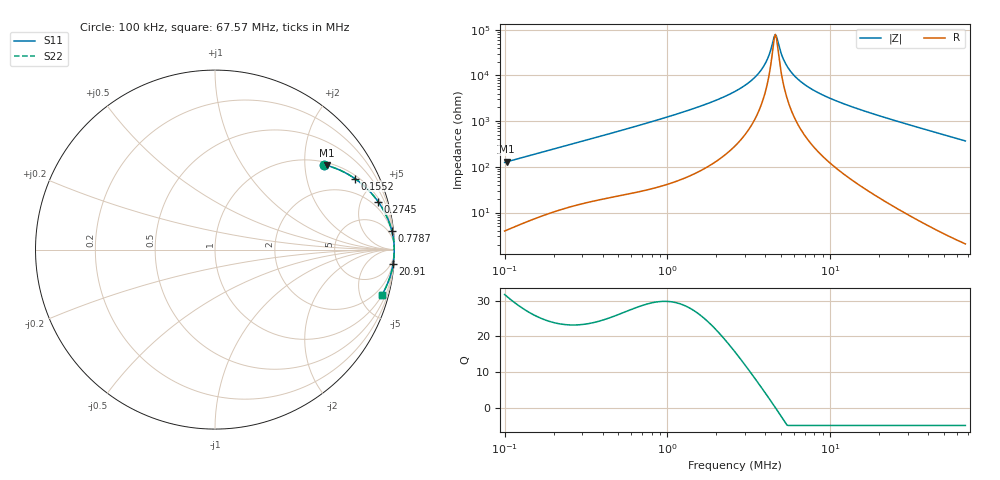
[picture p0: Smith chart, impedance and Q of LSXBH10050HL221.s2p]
! LSXBH10050HL221  S-PARAMETER MODEL  ( General Type )
! Model Generated by TAIYO YUDEN Corporation (http://www.ty-top.com)
! Version 3.0
! TAIYO YUDEN Control No. 180118NI43SB-FBB
! Copyright(c) 2007 TAIYO YUDEN CO.,LTD. All Rights Reserved.
! Product Description (link to TY-COMPAS)
! https://ds.yuden.co.jp/TYCOMPAS/or/detail?pn=LSXBH10050HL221M&u=M
! Products Name : Inductors
! Characteristics :
!  Inductance : 220 uH , SRF(min) : 3 MHz , DC Resistance(max) : 0.585 Ohm
!  Rated Current : Saturation :1000 mA , Temp Rise : 800 mA (40 degC)
!  Case Size : 10.0 x 9.8 / 0.394 x 0.386 [mm/inch] , Thickness : 5 / 0.197 [mm/inch]
!  (Conditions: Temperature = 25 degC , DC Bias Current/Voltage = 0A / 0V)
! External Node Assignments :
!  1  o---GGG---o  2
! GND o---------o GND
! Frequency Range : 0.1MHz  -  67.570357MHz  [ 402 STEP ]
# MHz S RI R 50
! Freq[MHz].  S11 Real  S11 Imag  S21 Real  S21 Imag  S12 Real  S12 Imag  S22 Real  S22 Imag
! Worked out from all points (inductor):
!   401 points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, 100 kHz to 67.57 MHz, reference 50 ohm
!   read as one part in series: L = 198 uH near 103.3 kHz
!   highest Q = 31.2 at 103.3 kHz (marker M1), where L = 199 uH
!   self-resonance near 4.597 MHz
!   S11 on the Smith chart (normalised r, x): 100 kHz: 1.08, +2.51; 155.2 kHz: 1.15, +3.85; 274.5 kHz: 1.29, +6.69; 778.7 kHz: 2, +19; 20.91 MHz: 1, -25; 67.57 MHz: 1.04, -7.39
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0.1  0.608 0.4727  0.392 -0.4727  0.392 -0.4727  0.608 0.4727
0.103312  0.6226 0.469  0.3774 -0.469  0.3774 -0.469  0.6226 0.469
0.155242  0.779 0.3959  0.221 -0.3959  0.221 -0.3959  0.779 0.3959
0.274544  0.9084 0.2677  0.0916 -0.2677  0.0916 -0.2677  0.9084 0.2677
0.297841  0.92 0.2507  0.08 -0.2507  0.08 -0.2507  0.92 0.2507
0.778705  0.9855 0.1035  0.0145 -0.1035  0.0145 -0.1035  0.9855 0.1035
0.887091  0.9886 0.0905  0.0114 -0.0905  0.0114 -0.0905  0.9886 0.0905
2.59943  0.9981 0.0222  0.00192 -0.0222  0.00192 -0.0222  0.9981 0.0222
3.212515  0.9985 0.0135  0.00153 -0.0135  0.00153 -0.0135  0.9985 0.0135
3.719758  0.9986 0.0079  0.00137 -0.0079  0.00137 -0.0079  0.9986 0.0079
4.101673  0.9987 0.00425  0.0013 -0.00425  0.0013 -0.00425  0.9987 0.00425
4.449723  0.9987 0.00124  0.00127 -0.00124  0.00127 -0.00124  0.9987 0.00124
4.597077  0.9987 3.3e-05  0.00126 -3.3e-05  0.00126 -3.3e-05  0.9987 3.3e-05
4.74931  0.9987 -0.00117  0.00126 0.00117  0.00126 0.00117  0.9987 -0.00117
5.152316  0.9987 -0.00418  0.00127 0.00418  0.00127 0.00418  0.9987 -0.00418
5.589519  0.9987 -0.00723  0.00129 0.00723  0.00129 0.00723  0.9987 -0.00723
6.367509  0.9986 -0.0122  0.00138 0.0122  0.00138 0.0122  0.9986 -0.0122
7.742162  0.9984 -0.0201  0.00162 0.0201  0.00162 0.0201  0.9984 -0.0201
11.44584  0.9973 -0.0384  0.00268 0.0384  0.00268 0.0384  0.9973 -0.0384
20.91222  0.9924 -0.0793  0.00755 0.0793  0.00755 0.0793  0.9924 -0.0793
23.05932  0.9909 -0.0881  0.00905 0.0881  0.00905 0.0881  0.9909 -0.0881
67.57036  0.9306 -0.2513  0.0694 0.2513  0.0694 0.2513  0.9306 -0.2513
